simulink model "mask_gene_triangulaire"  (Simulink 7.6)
settings: Solver=ode15s  StartTime=0.0  StopTime=2  RelTol=1e-3
libraries: fl_lib x9, elec_lib x3, nesl_utility x3

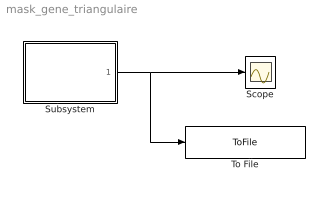
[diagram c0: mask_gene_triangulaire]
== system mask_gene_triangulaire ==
  Scope : Scope
  Subsystem : Subsystem
  To File : ToFile  Filename=signal_triangle  MatrixName=x
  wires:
  Subsystem/1(tri) -> Scope/1, To File/1

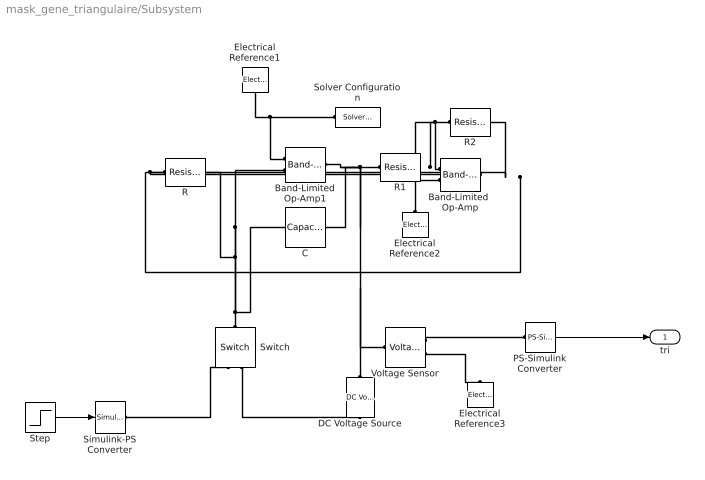
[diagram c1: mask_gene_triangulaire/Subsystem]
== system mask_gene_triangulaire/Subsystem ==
  Band-Limited  Op-Amp : elec_lib/Integrated Circuits/Band-Limited Op-Amp  DialogController=NetworkEngine.DynNeDlgSource  SystemSampleTime=-1  A=1000  Rin=1e+06 Ohm  Rout=100 Ohm  Vmin=-15 V  Vmax=15 V  Vdotmax=1000 V/s  f=1e+05 Hz  V0=0 V  LocalVarNames=|power  LocalVarDescs=|Dissipated power (W)  LocalVarLogging=0
  Band-Limited Op-Amp1 : elec_lib/Integrated Circuits/Band-Limited Op-Amp  DialogController=NetworkEngine.DynNeDlgSource  SystemSampleTime=-1  A=1000  Rin=1e+06 Ohm  Rout=100 Ohm  Vmin=-15 V  Vmax=15 V  Vdotmax=1000 V/s  f=1e+05 Hz  V0=0 V  LocalVarNames=|power  LocalVarDescs=|Dissipated power (W)  LocalVarLogging=0
  C : fl_lib/Electrical/Electrical Elements/Capacitor  DialogController=NetworkEngine.DynNeDlgSource  SystemSampleTime=-1  c=1e-6 F  v0=0 V  r=1e-6 Ohm  g=0 1/Ohm  i_Log=off  v_Log=off  vc_Log=off  LocalVarNames=|current|voltage|power  LocalVarDescs=|Capacitor current (A)|Voltage across capacitor (V)|Power (W)  LocalVarLogging=[0 0 0]
  DC Voltage Source : elec_lib/Additional Components/SPICE-Compatible Components/Sources/DC Voltage Source  DialogController=NetworkEngine.DynNeDlgSource  SystemSampleTime=-1  DC=1 V  current_Log=off  voltage_Log=off  power_Log=off  LocalVarNames=|current|voltage|power  LocalVarDescs=|Current (A)|Voltage (V)|Power (W)  LocalVarLogging=[0 0 0]
  Electrical Reference1 : fl_lib/Electrical/Electrical Elements/Electrical Reference  DialogController=NetworkEngine.DynNeDlgSource  SystemSampleTime=-1  i_Log=off  LocalVarNames=|i  LocalVarDescs=|i  LocalVarLogging=[]
  Electrical Reference2 : fl_lib/Electrical/Electrical Elements/Electrical Reference  DialogController=NetworkEngine.DynNeDlgSource  SystemSampleTime=-1  i_Log=off  LocalVarNames=|i  LocalVarDescs=|i  LocalVarLogging=[]
  Electrical Reference3 : fl_lib/Electrical/Electrical Elements/Electrical Reference  DialogController=NetworkEngine.DynNeDlgSource  SystemSampleTime=-1  i_Log=off  LocalVarNames=|i  LocalVarDescs=|i  LocalVarLogging=[]
  PS-Simulink Converter : nesl_utility/PS-Simulink Converter  DialogController=NetworkEngine.DynNeUtilDlgSource  SystemSampleTime=-1  PhysicalDomain=network_engine_domain  LeftPortType=input  RightPortType=output  SubClassName=ps_output  Unit=1  AffineConversion=off
  R : fl_lib/Electrical/Electrical Elements/Resistor  DialogController=NetworkEngine.DynNeDlgSource  SystemSampleTime=-1  R=100e3 Ohm  i_Log=off  v_Log=off  LocalVarNames=|current|voltage|power  LocalVarDescs=|Resistor current (A)|Voltage across resistor (V)|Power (W)  LocalVarLogging=[0 0 0]
  R1 : fl_lib/Electrical/Electrical Elements/Resistor  DialogController=NetworkEngine.DynNeDlgSource  SystemSampleTime=-1  R=10e3 Ohm  i_Log=off  v_Log=off  LocalVarNames=|current|voltage|power  LocalVarDescs=|Resistor current (A)|Voltage across resistor (V)|Power (W)  LocalVarLogging=[0 0 0]
  R2 : fl_lib/Electrical/Electrical Elements/Resistor  DialogController=NetworkEngine.DynNeDlgSource  SystemSampleTime=-1  R=10e3 Ohm  i_Log=off  v_Log=off  LocalVarNames=|current|voltage|power  LocalVarDescs=|Resistor current (A)|Voltage across resistor (V)|Power (W)  LocalVarLogging=[0 0 0]
  Simulink-PS Converter : nesl_utility/Simulink-PS Converter  DialogController=NetworkEngine.DynNeUtilDlgSource  SystemSampleTime=-1  PhysicalDomain=network_engine_domain  LeftPortType=input  RightPortType=output  SubClassName=ps_input  Unit=1  AffineConversion=off  InputFilterTimeConstant=.001  UdotUserProvided=0
  Solver Configuration : nesl_utility/Solver Configuration  DialogController=NetworkEngine.DynNeUtilDlgSource  SystemSampleTime=-1  PhysicalDomain=network_engine_domain  LeftPortType=input  RightPortType=generic  SubClassName=solver  Accelerate=off  Profile=off  ResidualTolerance=1e-9  MaxNonlinIter=12  MaxModeIter=2  DoFixedCost=off  UseLocalSampling=off  DoDC=off  LinearAlgebra=Sparse  LocalSolverSampleTime=.001  LocalSolverChoice=NE_BACKWARD_EULER_ADVANCER  UseLocalSolver=off
  Step : Step  Time=0  Before=0.1  After=0  SampleTime=0
  Switch : fl_lib/Electrical/Electrical Elements/Switch  DialogController=NetworkEngine.DynNeDlgSource  SystemSampleTime=-1  R_closed=0.01 Ohm  G_open=1e-08 1/Ohm  Threshold=0  i_Log=off  v_Log=off  LocalVarNames=|i|v  LocalVarDescs=|i|v  LocalVarLogging=[0 0]
  Voltage Sensor : fl_lib/Electrical/Electrical Sensors/Voltage Sensor  DialogController=NetworkEngine.DynNeDlgSource  SystemSampleTime=-1  i1_Log=off  v1_Log=off  LocalVarNames=|i1|v1  LocalVarDescs=|i1|v1  LocalVarLogging=[]
  tri : Outport
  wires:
  PS-Simulink Converter/1 -> tri/1
  Step/1 -> Simulink-PS Converter/1
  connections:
  Simulink-PS Converter/RConn1 -- Switch/RConn1
  Voltage Sensor/RConn1 -- PS-Simulink Converter/LConn1
  Switch/RConn2 -- DC Voltage Source/RConn1
  Band-Limited Op-Amp1/RConn1 -- DC Voltage Source/LConn1 -- Voltage Sensor/LConn1 -- C/RConn1 -- R1/LConn1
  Switch/LConn1 -- Band-Limited Op-Amp1/LConn2 -- R/RConn1 -- C/LConn1
  Solver Configuration/RConn1 -- Band-Limited Op-Amp1/LConn1 -- Electrical Reference1/LConn1
  R/LConn1 -- Band-Limited  Op-Amp/RConn1 -- R2/RConn1
  Electrical Reference2/LConn1 -- Band-Limited  Op-Amp/LConn2
  R2/LConn1 -- Band-Limited  Op-Amp/LConn1 -- R1/RConn1
  Voltage Sensor/RConn2 -- Electrical Reference3/LConn1
